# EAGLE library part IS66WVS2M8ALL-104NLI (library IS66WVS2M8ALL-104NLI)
SRAM 16Mb, SerialRAM, 1.65V-1.95V, 104MHz, 8 pin SOIC 150 mil, RoHS Source: Datasheet
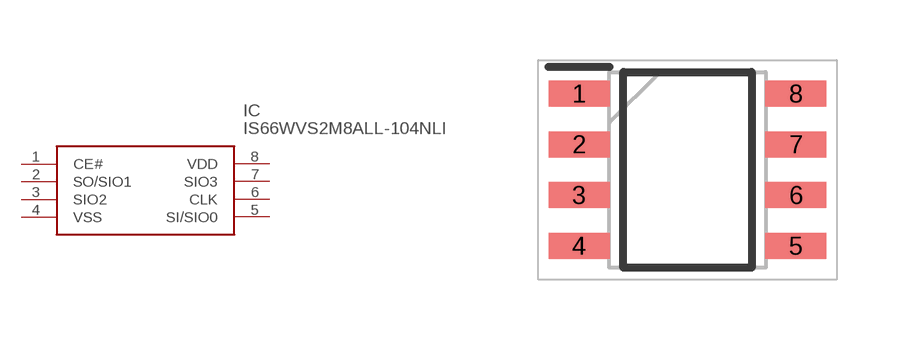
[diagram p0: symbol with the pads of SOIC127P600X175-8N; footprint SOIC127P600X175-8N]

Designator prefix IC

## IS66WVS2M8ALL-104NLI (Description: SRAM 16Mb, SerialRAM, 1.65V-1.95V, 104MHz, 8 pin SOIC 150 mil, RoHS; Height: 1.75mm; Manufacturer_Name: Integrated Silicon Solution Inc.; Manufacturer_Part_Number: IS66WVS2M8ALL-104NLI)  [SOIC127P600X175-8N]
1  CE#
2  SO/SIO1
3  SIO2
4  VSS
5  SI/SIO0
6  CLK
7  SIO3
8  VDD

## Footprint SOIC127P600X175-8N (pad centres in mm)
10.2 8-PIN JEDEC 150MIL BROAD SMALL OUTLINE INTEGRATED CIRCUIT (SOIC) PACKAGE (N)
smd 1.525 x 0.65: 1 -2.712,1.905; 2 -2.712,0.635; 3 -2.712,-0.635; 4 -2.712,-1.905; 5 2.712,-1.905; 6 2.712,-0.635; 7 2.712,0.635; 8 2.712,1.905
